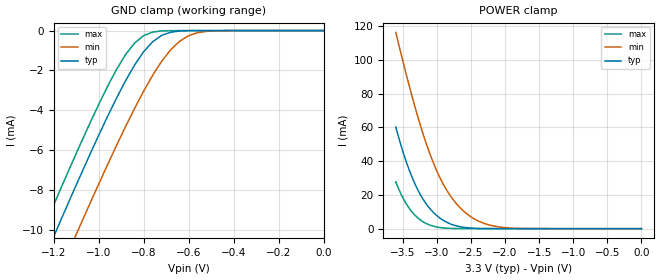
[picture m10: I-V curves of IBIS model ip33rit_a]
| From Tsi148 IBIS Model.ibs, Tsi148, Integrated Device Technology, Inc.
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|   MODEL ip33rit_a
[Model]   ip33rit_a
Model_type   Input
Vinl  = 0.8V
Vinh  = 2.0V
|   typ   min   max
C_comp   0.63pF   0.58pF  0.67pF
[Temperature Range]   50.00   125.00   0.00
[Voltage Range]   3.300   3.000   3.600
|   typ   min   max
|[Supply]   VDD   1.80   1.65   1.95
|[Supply]   VDD330   3.30   3.00   3.60
[Add Submodel]
| Submodel Name   Mode
Up.ip33rit_a   Non-Driving
Dn.ip33rit_a   Non-Driving
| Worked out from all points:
|   GND clamp passes 1 mA (typ) near -0.80 V on its own axis
|   POWER clamp passes 1 mA (typ) near -2.63 V on its own axis
[POWER_Clamp]   | Note: Vtable = Vcc - Vout
| Voltage   I(typ)   I(min)   I(max)
-3.6V     60.2mA     116.3mA    27.69mA
-3.48V    43.67mA    96.64mA    17.04mA
-3.36V    30.3mA     78.14mA    9.798mA
-3.24V    20.18mA    61.24mA    5.162mA
-3.08V    10.92mA    42.12mA    1.825mA
-2.96V    6.444mA    30.76mA    703uA
-2.84V    3.523mA    21.89mA    233uA
-2.72V    1.75mA     15.16mA    70uA
-2.56V    578uA      8.808mA    13uA
-2.32V    80uA       3.344mA    1uA
-2V       5uA        606uA      0A
0V        0A         0A         0A
[GND_Clamp]   | Note: Vtable = Vout
| Voltage   I(typ)   I(min)   I(max)
-3.6V     -76.49mA   -78.79mA   -75.06mA
-1.28V    -12.45mA   -14.94mA   -10.87mA
-1.24V    -11.4mA    -13.88mA   -9.809mA
-1.2V     -10.35mA   -12.84mA   -8.759mA
-1.12V    -8.273mA   -10.76mA   -6.689mA
-1.08V    -7.253mA   -9.729mA   -5.675mA
-920mV    -3.381mA   -5.752mA   -1.944mA
-840mV    -1.725mA   -3.901mA   -626uA
-760mV    -561uA     -2.244mA   -74uA
-640mV    -23uA      -536uA     -1uA
-520mV    0A         -38uA      0A
0V        0A         0A         0A
